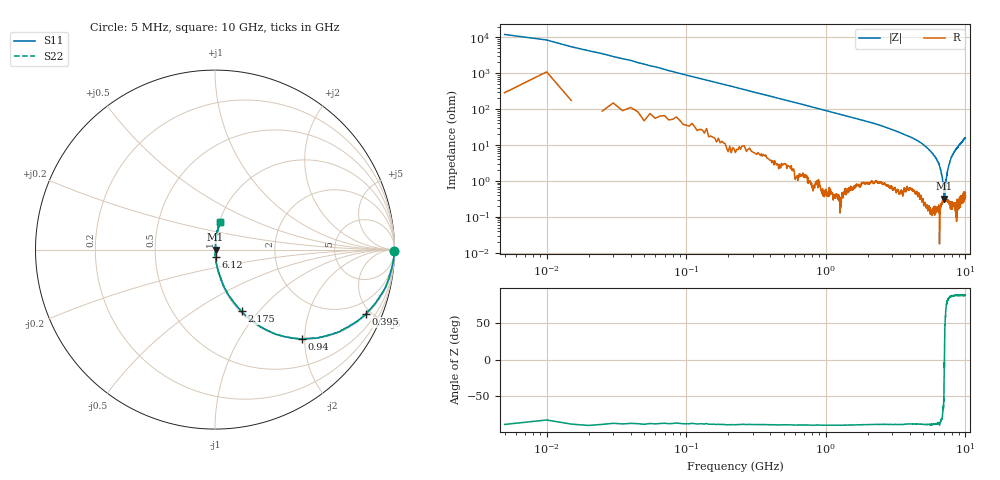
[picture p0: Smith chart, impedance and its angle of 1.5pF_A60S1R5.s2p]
! Amotech Co.,Ltd.
! http://www.amotech.co.kr/
! Part Number: A60S1R5
! These Parameters are Measured in Series Mode Connection
! Operation Temp=25[degC], DC Bias Voltage=0[V]
! Freq. Start=5[MHz] Stop=10[GHz], 2000[Steps]
! Date: Monday, July 13, 2020, 01:50:22
# GHZ S RI R 50.000000
!Freq.(Hz) S11(Real) S11(Imag) S21(Real) S21(Imag) S12(Real) S12(Imag) S22(Real) S22(Imag)
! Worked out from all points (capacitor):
!   2000 points, 5 MHz to 10 GHz, reference 50 ohm
!   read as one part in series: C = 1.79 pF near 55 MHz
!   lowest |Z| = 319 mohm at 7.075 GHz (marker M1)
!   series resonance near 7.074 GHz, so ESL is about 280 pH
!   S11 on the Smith chart (normalised r, x): 5 MHz: open; 395 MHz: 1.08, -4.65; 940 MHz: 1.01, -1.94; 2.175 GHz: 1.02, -0.81; 6.12 GHz: 1.00, -0.09; 10 GHz: 1.01, +0.32
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0.005  0.9997 -0.00832  0.000268 0.00832  0.000268 0.00832  0.9997 -0.00832
0.07  0.99 -0.0769  0.00999 0.0769  0.00999 0.0769  0.99 -0.0769
0.125  0.9756 -0.1362  0.0244 0.1362  0.0244 0.1362  0.9756 -0.1362
0.235  0.9334 -0.2398  0.0666 0.2398  0.0666 0.2398  0.9334 -0.2398
0.395  0.8397 -0.3587  0.1603 0.3587  0.1603 0.3587  0.8397 -0.3587
0.625  0.6814 -0.4611  0.3186 0.4611  0.3186 0.4611  0.6814 -0.4611
0.94  0.4851 -0.4975  0.5149 0.4975  0.5149 0.4975  0.4851 -0.4975
1.675  0.2288 -0.413  0.7712 0.413  0.7712 0.413  0.2288 -0.413
2.175  0.1477 -0.344  0.8523 0.344  0.8523 0.344  0.1477 -0.344
3.34  0.053 -0.2139  0.947 0.2139  0.947 0.2139  0.053 -0.2139
5.005  0.0128 -0.1007  0.9872 0.1007  0.9872 0.1007  0.0128 -0.1007
6.12  0.00359 -0.0428  0.9964 0.0428  0.9964 0.0428  0.00359 -0.0428
6.42  0.00282 -0.0316  0.9972 0.0316  0.9972 0.0316  0.00282 -0.0316
6.67  0.00242 -0.0194  0.9976 0.0194  0.9976 0.0194  0.00242 -0.0194
6.84  0.0028 -0.0118  0.9972 0.0118  0.9972 0.0118  0.0028 -0.0118
7.075  0.00318 0.000109  0.9968 -0.000109  0.9968 -0.000109  0.00318 0.000109
7.15  0.00272 0.00322  0.9973 -0.00322  0.9973 -0.00322  0.00272 0.00322
7.275  0.00328 0.0105  0.9967 -0.0105  0.9967 -0.0105  0.00328 0.0105
7.455  0.00332 0.0192  0.9967 -0.0192  0.9967 -0.0192  0.00332 0.0192
7.91  0.00439 0.0444  0.9956 -0.0444  0.9956 -0.0444  0.00439 0.0444
8.335  0.0061 0.0641  0.9939 -0.0641  0.9939 -0.0641  0.0061 0.0641
10  0.0282 0.155  0.9718 -0.155  0.9718 -0.155  0.0282 0.155
